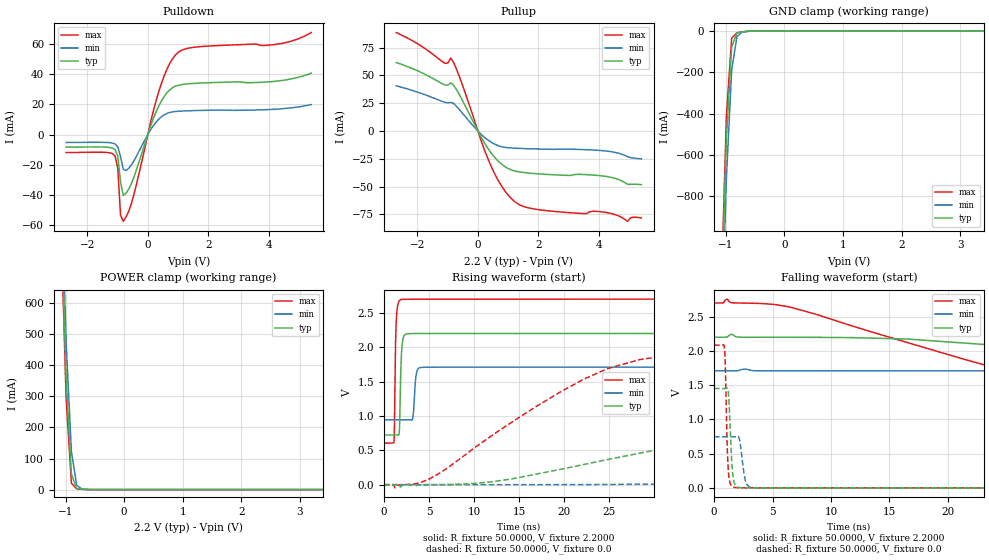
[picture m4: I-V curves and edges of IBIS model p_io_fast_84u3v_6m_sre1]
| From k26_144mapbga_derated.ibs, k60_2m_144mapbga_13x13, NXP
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[Model] p_io_fast_84u3v_6m_sre1
|   Model p_io_fast_84u3v_6m_sre1
| Library cells for typ/min/max conditions are connected as defined below:
|  pad - External Pad
|  ipp_do - Core Input
|  ipp_obe - Output Buffer Enable
|  esd_boost - vdd_s_3v
|  esd_bus - vdd_s_3v
|  ipp_ina40a_3v - NC
|  ipp_ina40b_3v - NC
|  ipp_ina_3v - NC
|  ipp_ind - NC
|  ipp_ind_3v - NC
|  ipp_sre - vdd_s_lv
|  vdd_s_3v - vdd_s_3v
|  vdd_s_lv - vdd_s_lv
|  vss_bulk - vss_bulk
|  vss_s_lv - vss_s_lv
| All other pins connected to ground
Model_type I/O
Polarity   Non-Inverting
Enable   Active-High
Vinl =   0.6600V
Vinh =   1.6500V
Vmeas =  1.1000V
Cref =   25.0000pF
Rref =   50.0000
Vref =   0.0V
C_comp   2.4452pF   2.2297pF   2.7119pF
[Temperature Range]   25.0000   0.1250k   -40.0000
[Voltage Range]   2.2000V   1.7100V   2.7000V
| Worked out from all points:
|   slope of the pulldown table from 0 to 0.33 V, typ, clamps not added: 18.9 ohm
|   slope of the pullup table from 0 to 0.33 V, typ, clamps not added: 21.2 ohm
|   GND clamp passes 1 mA (typ) near -0.55 V on its own axis
|   POWER clamp passes 1 mA (typ) near -0.72 V on its own axis
|   rising waveform, R_fixture 50.0000, V_fixture 2.2000: 20-80 % time 180ps typ, 232ps min, 157ps max; typ from 0.723 V to 2.2 V
|   rising waveform, R_fixture 50.0000, V_fixture 0.0: 20-80 % time 39.1ns typ, 105ns min, 15.6ns max; typ from 0 V to 1.45 V
|   falling waveform, R_fixture 50.0000, V_fixture 2.2000: 20-80 % time 65.9ns typ, 155ns min, 29.6ns max; typ from 2.2 V to 0.723 V
|   falling waveform, R_fixture 50.0000, V_fixture 0.0: 20-80 % time 240ps typ, 348ps min, 185ps max; typ from 1.45 V to 0 V
[Pulldown]
|Voltage   I(typ)   I(min)   I(max)
-2.7V     -8.31mA    -5.23mA    -11.88mA
-1.08V    -9.994mA   -6.229mA   -14.18mA
-990mV    -14.38mA   -8.172mA   -22.36mA
-900mV    -31.61mA   -14.63mA   -53.43mA
-810mV    -40.21mA   -22.92mA   -57.28mA
-540mV    -32.32mA   -19.93mA   -45.49mA
360mV     18.77mA    10.12mA    28.27mA
630mV     27.55mA    13.96mA    43.04mA
900mV     31.86mA    15.23mA    52.31mA
1.62V     33.93mA    15.9mA     57.87mA
4.32V     35.46mA    16.9mA     59.88mA
5.4V      40.6mA     19.8mA     67.4mA
[Pullup]
|Voltage   I(typ)   I(min)   I(max)
-2.7V     61.6mA     40.7mA     88.6mA
-1.08V    41.41mA    25.81mA    60.81mA
-900mV    43.32mA    25.75mA    65.7mA
-630mV    33.56mA    19.89mA    50.33mA
180mV     -9.091mA   -4.822mA   -14.35mA
450mV     -20.18mA   -10.26mA   -32.51mA
810mV     -30.38mA   -14.27mA   -50.71mA
1.26V     -36.2mA    -15.46mA   -64.37mA
2.25V     -38.95mA   -16.35mA   -71.56mA
4.14V     -40.49mA   -17.71mA   -72.91mA
4.95V     -47.96mA   -23.1mA    -81.2mA
5.4V      -48.23mA   -25.1mA    -78.16mA
[GND_clamp]
|Voltage   I(typ)   I(min)   I(max)
-2.7V     -21.84A    -21.72A    -21.97A
-1.08V    -1.363A    -1.529A    -1.277A
-990mV    -526.3mA   -714.4mA   -415.1mA
-900mV    -78.38mA   -191.9mA   -35.01mA
-810mV    -10.19mA   -27.77mA   -9.384mA
-720mV    -4.846mA   -5.816mA   -5.628mA
-450mV    -161.5uA   -306uA     -96.62uA
5.4V      0A         0A         0A
[POWER_clamp]
|Voltage   I(typ)   I(min)   I(max)
-2.7V     13.99A     13.91A     14.09A
-1.08V    915.5mA    1.013A     866mA
-990mV    361.3mA    476.1mA    293mA
-900mV    49.95mA    121.8mA    20.75mA
-810mV    3.622mA    14.14mA    2.341mA
-720mV    938.4uA    1.525mA    905uA
-540mV    64.25uA    64.25uA    24.86uA
5.4V      0A         0A         0A
[Ramp]
| variable   typ   min   max
dV/dt_r  0.8705/39.0713n   0.4471/0.1053u   1.2508/15.6028n
dV/dt_f  0.8860/65.9047n   0.4526/0.1546u   1.2570/29.5991n
R_load = 50.0000
[Rising Waveform]
R_fixture= 50.0000
V_fixture= 2.2000
V_fixture_min= 1.7100
V_fixture_max= 2.7000
|time   V(typ)   V(min)   V(max)
0s        723.3mV    944.3mV    605mV
1.111ns   723.3mV    944.3mV    619.7mV
1.267ns   723.3mV    944.3mV    1.937V
1.379ns   723.4mV    944.3mV    2.417V
1.726ns   828mV      944.3mV    2.679V
2.032ns   2.052V     944.2mV    2.697V
3.13ns    2.199V     942mV      2.699V
3.663ns   2.199V     1.651V     2.699V
4.859ns   2.2V       1.709V     2.699V
500ns     2.2V       1.71V      2.7V
[Rising Waveform]
R_fixture= 50.0000
V_fixture= 0.0
V_fixture_min= 0.0
V_fixture_max= 0.0
|time   V(typ)   V(min)   V(max)
0s        1.4nV      47.93nV    52.08pV
4.997ns   30.94uV    -486.8uV   80.9mV
16.79ns   151.3mV    201uV      1.13V
24.81ns   365.7mV    3.045mV    1.689V
33.05ns   579.6mV    10.19mV    1.912V
45.27ns   870.3mV    45.91mV    2.02V
77.53ns   1.321V     201.1mV    2.079V
109.1ns   1.414V     365.5mV    2.084V
234.4ns   1.45V      694mV      2.085V
500ns     1.451V     745.2mV    2.085V
[Falling Waveform]
R_fixture= 50.0000
V_fixture= 2.2000
V_fixture_min= 1.7100
V_fixture_max= 2.7000
|time   V(typ)   V(min)   V(max)
0s        2.2V       1.71V      2.7V
6.43ns    2.2V       1.71V      2.644V
24.59ns   2.071V     1.71V      1.727V
40.58ns   1.82V      1.706V     1.085V
48.9ns    1.686V     1.7V       877.3mV
68.81ns   1.385V     1.665V     683mV
100.7ns   1.022V     1.569V     622.1mV
149.2ns   800.7mV    1.401V     606.2mV
285ns     726.3mV    1.066V     605mV
500ns     723.3mV    955.7mV    605mV
[Falling Waveform]
R_fixture= 50.0000
V_fixture= 0.0
V_fixture_min= 0.0
V_fixture_max= 0.0
|time   V(typ)   V(min)   V(max)
0s        1.451V     745.8mV    2.085V
882.1ps   1.45V      745.8mV    2.058V
951.4ps   1.45V      745.8mV    1.857V
1.146ns   1.451V     745.8mV    490.9mV
1.244ns   1.348V     745.8mV    203mV
1.583ns   220.2mV    745.1mV    17.9mV
2.045ns   8.288mV    756.1mV    1.151mV
2.796ns   950uV      51.55mV    1.04mV
3.74ns    264.8uV    561.2uV    250uV
500ns     525.1nV    -844.6nV   452.6pV
